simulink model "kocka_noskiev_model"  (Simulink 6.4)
settings: Solver=ode45  StartTime=0.0  StopTime=10  RelTol=1e-3
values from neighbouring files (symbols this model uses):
  A = [0 1 0 0 0    [kockaLQG.m]    (also in kockaLQR.m; podklad.m = [dh1_h10 dh1_h20 0; testx.m = [ -0.195 0.195; 0.195 -0.205]; kulicka_na_tyci_LQG_podklad.m = [0 0;1 0])
  B = [0    [kockaLQG.m]    (also in kockaLQR.m; podklad.m = [dh1_q0; testx.m = [0.0047; 0]; kulicka_na_tyci_LQG_podklad.m = [7.14;0])
  C = [1 0 0 0 0]    [kockaLQG.m]    (also in kockaLQR.m; podklad.m = [0 0 1]; testx.m = [0 1]; kulicka_na_tyci_LQG_podklad.m = [0 1])

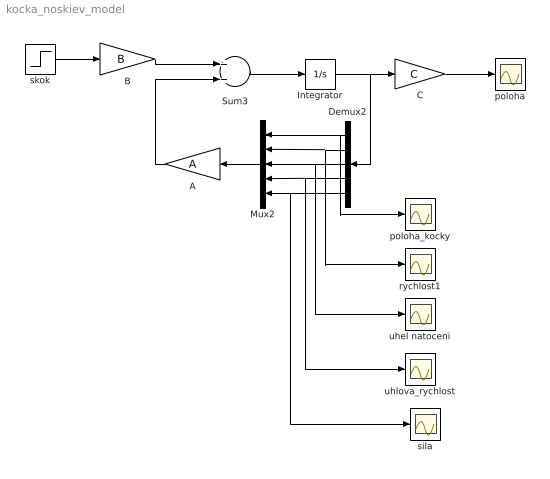
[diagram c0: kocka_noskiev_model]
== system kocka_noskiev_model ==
  A : Gain  Orientation=left  Gain=A  Multiplication=Matrix(K*u)
  B : Gain  Gain=B  Multiplication=Matrix(K*u)
  C : Gain  Gain=C  Multiplication=Matrix(K*u)
  Demux2 : Demux  Orientation=left  Outputs=5
  Integrator : Integrator
  Mux2 : Mux  Orientation=left  Inputs=5
  Sum3 : Sum
  poloha : Scope
  poloha_kocky : Scope
  rychlost1 : Scope
  sila : Scope
  skok : Step  Time=0  SampleTime=0
  uhel natoceni : Scope
  uhlova_rychlost : Scope
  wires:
  Sum3/1 -> Integrator/1
  Integrator/1 -> Demux2/1, C/1
  Demux2/1 -> poloha_kocky/1, Mux2/1
  Demux2/2 -> rychlost1/1, Mux2/2
  Demux2/3 -> uhel natoceni/1, Mux2/3
  Demux2/4 -> uhlova_rychlost/1, Mux2/4
  Mux2/1 -> A/1
  A/1 -> Sum3/2
  B/1 -> Sum3/1
  skok/1 -> B/1
  C/1 -> poloha/1
  Demux2/5 -> Mux2/5, sila/1
